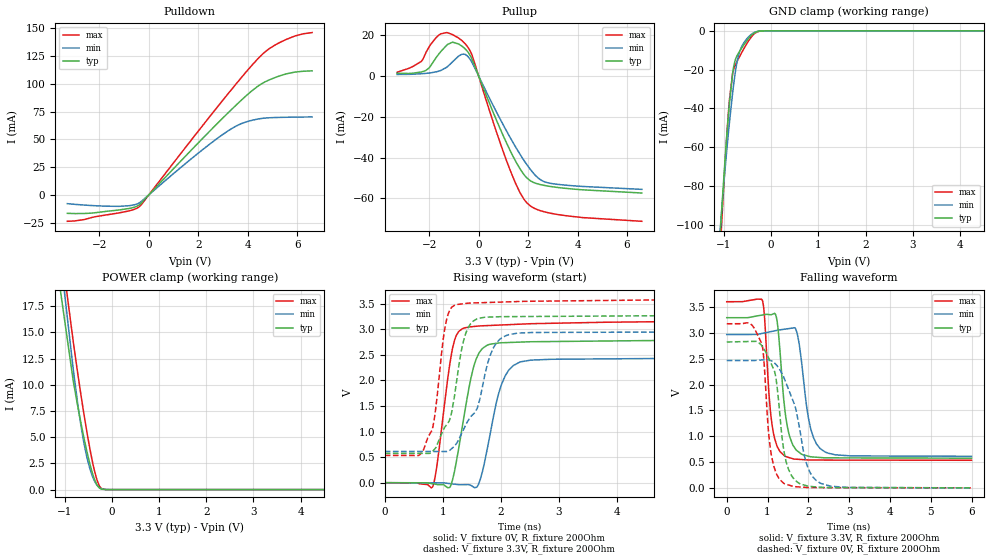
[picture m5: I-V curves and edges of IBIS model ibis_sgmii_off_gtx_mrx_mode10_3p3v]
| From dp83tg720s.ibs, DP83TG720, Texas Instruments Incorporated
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| ibis_sgmii_off_gtx_mrx_mode10_3p3v
[Model]   ibis_sgmii_off_gtx_mrx_mode10_3p3v
Model_type   I/O
Polarity   Non-Inverting
Enable   Active-Low
Vinl = 0.99
Vinh = 2.31
Vmeas = 1.65
Vref = 1.65
Cref = 2pF
Rref = 100000
|   typ   min   max
C_comp   3.97pF   3.92pF   4.02pF
[Voltage Range]   3.3   2.97   3.63
[Temperature Range]   27   150   -40
[Pullup Reference]   3.3   2.97   3.63
[Pulldown Reference]   -0   -0   0
[Power Clamp Reference]   3.3   2.97   3.63
[GND Clamp Reference]   0   0   0
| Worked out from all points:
|   slope of the pulldown table from 0 to 0.495 V, typ, clamps not added: 42.2 ohm
|   slope of the pullup table from 0 to 0.495 V, typ, clamps not added: 32.8 ohm
|   GND clamp passes 1 mA (typ) near -0.35 V on its own axis
|   POWER clamp passes 1 mA (typ) near -0.37 V on its own axis
|   falling waveform, V_fixture 3.3V, R_fixture 200Ohm: 20-80 % time 209ps typ, 257ps min, 174ps max; typ from 3.29 V to 0.575 V
|   rising waveform, V_fixture 0V, R_fixture 200Ohm: 20-80 % time 268ps typ, 288ps min, 218ps max; typ from 0 V to 2.8 V
|   rising waveform, V_fixture 3.3V, R_fixture 200Ohm: 20-80 % time 297ps typ, 441ps min, 192ps max; typ from 0.575 V to 3.28 V
|   falling waveform, V_fixture 0V, R_fixture 200Ohm: 20-80 % time 270ps typ, 464ps min, 190ps max; typ from 2.82 V to 0 V
[Pulldown]
|   Voltage   I(typ)   I(min)   I(max)
-3.3V     -16.73mA   -7.996mA   -23.91mA
-2.33V    -16.53mA   -9.677mA   -20.61mA
-1.211V   -13.7mA    -10.43mA   -16.35mA
-676.5mV  -11.73mA   -9.433mA   -13.76mA
-399.3mV  -9.238mA   -7.464mA   -10.89mA
2.234V    52.23mA    41.75mA    64.12mA
3.046V    70.46mA    55.28mA    86.81mA
3.59V     82.23mA    62.68mA    101.7mA
4.412V    98.01mA    68.33mA    122.8mA
4.887V    103.8mA    69.47mA    132.1mA
5.877V    110.5mA    70mA       143mA
6.6V      111.8mA    70.21mA    146.3mA
[GND Clamp]
|   Voltage   I(typ)   I(min)   I(max)
-3.3V     -1.085A    -934.6mA   -1.211A
-1.092V   -110.2mA   -106.5mA   -119.2mA
-1.063V   -98.5mA    -97.09mA   -105.8mA
-1.053V   -94.66mA   -94.01mA   -101.4mA
-963.6mV  -61.91mA   -67.88mA   -63.46mA
-904.2mV  -42.96mA   -52.32mA   -41.79mA
-815.1mV  -21.71mA   -31.82mA   -21.8mA
-726mV    -13mA      -16.49mA   -16mA
-646.8mV  -9.719mA   -9.375mA   -12.28mA
-488.4mV  -4.237mA   -3.373mA   -5.539mA
-330mV    -723.2uA   -565.9uA   -1.02mA
6.6V      0A         0A         0A
[Pullup]
|   Voltage   I(typ)   I(min)   I(max)
-3.3V     1.293mA    748.4uA    1.811mA
-2.33V    1.941mA    1.084mA    7.036mA
-2.142V   2.672mA    1.267mA    11.2mA
-1.538V   11.87mA    2.646mA    20.62mA
-1.053V   16.6mA     6.951mA    20.28mA
-815.1mV  15.72mA    9.702mA    18.66mA
-537.9mV  13.21mA    10.52mA    15.72mA
-280.5mV  8.591mA    6.894mA    10.64mA
1.125V    -32.76mA   -26.91mA   -41.43mA
1.957V    -50.09mA   -43.61mA   -62.32mA
2.788V    -53.99mA   -52.38mA   -67.04mA
6.6V      -57.42mA   -55.64mA   -71.3mA
[POWER Clamp]
|   Voltage   I(typ)   I(min)   I(max)
-3.3V     317.9mA    237mA      400.5mA
-1.181V   21.99mA    25.93mA    26.78mA
-815.1mV  10.35mA    11.45mA    14.1mA
-656.7mV  6.45mA     6.234mA    9.162mA
-587.4mV  4.9mA      4.403mA    7.158mA
-528mV    3.668mA    3.117mA    5.537mA
-458.7mV  2.373mA    1.935mA    3.791mA
-369.6mV  1.032mA    856.8uA    1.866mA
-310.2mV  435.4uA    402.5uA    888uA
-231mV    77.38uA    103.3uA    169.6uA
-72.6mV   430.8nA    2.491uA    462.9nA
6.6V      0A         0A         0A
[Ramp]
R_load = 200
|   typ   min   max
dV/dt_r   1.6783/2.67705e-10   1.46447/2.86317e-10   1.89874/2.17641e-10
dV/dt_f   1.63196/2.0849e-10   1.4141/2.54422e-10   1.84187/1.73954e-10
[Falling Waveform]
V_fixture = 3.3V
V_fixture_min = 2.97V
V_fixture_max = 3.63V
R_fixture = 200Ohm
C_fixture = 0F
|   Time   V(typ)   V(min)   V(max)
0s        3.295V     2.968V     3.604V
875.2ps   3.348V     2.992V     3.629V
1.111ns   3.359V     3.03V      1.224V
1.239ns   3.204V     3.051V     796.7mV
1.415ns   1.582V     3.072V     619.4mV
1.522ns   1.054V     3.084V     588.2mV
1.703ns   733.1mV    3.051V     554.9mV
2.052ns   602.7mV    1.165V     538.6mV
2.412ns   581.4mV    694.5mV    538.3mV
6ns       575mV      611.5mV    534.5mV
[Rising Waveform]
V_fixture = 0V
V_fixture_min = 0V
V_fixture_max = 0V
R_fixture = 200Ohm
C_fixture = 0F
|   Time   V(typ)   V(min)   V(max)
0s        60.13uV    67.26uV    83.75uV
822.8ps   -20.35mV   -2.073mV   -86.29mV
899.9ps   -35.23mV   -2.274mV   337.5mV
1.135ns   -62.17mV   -19.54mV   2.415V
1.338ns   1.102V     -39.58mV   3.013V
1.481ns   2.021V     -51.38mV   3.051V
1.63ns    2.546V     8.374mV    3.067V
2.001ns   2.738V     1.88V      3.086V
2.322ns   2.751V     2.356V     3.102V
6ns       2.797V     2.441V     3.165V
[Rising Waveform]
V_fixture = 3.3V
V_fixture_min = 2.97V
V_fixture_max = 3.63V
R_fixture = 200Ohm
C_fixture = 0F
|   Time   V(typ)   V(min)   V(max)
0s        574.7mV    611.3mV    534.3mV
662.2ps   573.7mV    610.8mV    629.2mV
845.2ps   639.8mV    610.6mV    1.186V
1.062ns   1.128V     610.5mV    3.17V
1.21ns    1.755V     728.1mV    3.478V
1.354ns   2.756V     1.03V      3.502V
1.475ns   3.101V     1.279V     3.515V
1.861ns   3.243V     2.609V     3.529V
2.109ns   3.249V     2.886V     3.538V
6ns       3.276V     2.951V     3.592V
[Falling Waveform]
|Gnd
V_fixture = 0V
V_fixture_min = 0V
V_fixture_max = 0V
R_fixture = 200Ohm
C_fixture = 0F
|   Time   V(typ)   V(min)   V(max)
0s        2.824V     2.465V     3.177V
575ps     2.835V     2.465V     3.18V
861ps     2.749V     2.477V     2.791V
1.086ns   2.412V     2.463V     673.2mV
1.21ns    2.107V     2.386V     284.9mV
1.393ns   761.6mV    2.152V     90.61mV
1.588ns   236.9mV    1.762V     38.23mV
1.982ns   36.87mV    407.3mV    7.362mV
2.286ns   13.67mV    94.1mV     4.744mV
6ns       292uV      292.5uV    267.8uV
